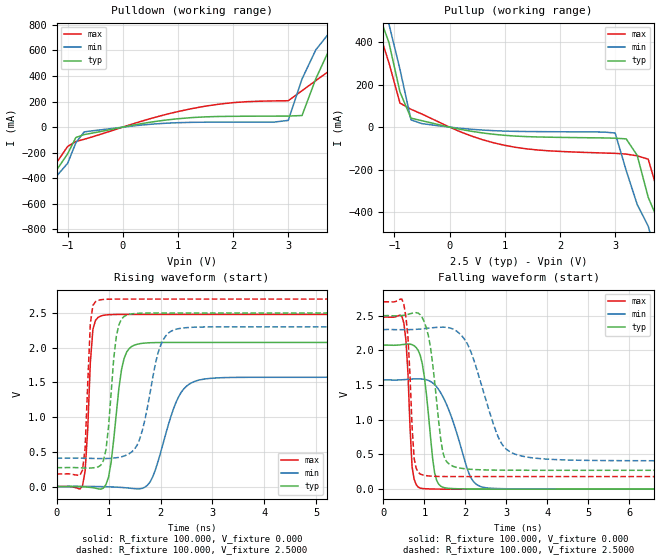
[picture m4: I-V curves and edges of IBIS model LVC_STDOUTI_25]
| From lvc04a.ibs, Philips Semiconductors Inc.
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|   Model LVC_STDOUTI_25
[Model]   LVC_STDOUTI_25
Model_type   Output
Polarity   Inverting
Vmeas =   1.25000V
Cref  =  50.0000pF
Rref  =   0.5000k
Vref  =   0.000V
C_comp   2.82pF   1.84pF   3.60pF
[Model Spec]
| Note: The input and output voltage ratings may be exceeded if the input and
|   output current ratings are observed (please refer to the data sheet)
|   Subparameter   typ   min   max
| Timing Thresholds
Vmeas   1.25   1.15   1.5
|Ambient temperature:   25.0000   85.0000   -40.0000
[Temperature Range]   35.0000   95.0000   -30.0000
[Voltage Range]   2.5000V   2.3000V   2.7000V
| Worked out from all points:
|   slope of the pulldown table from 0 to 0.375 V, typ, clamps not added: 12.6 ohm
|   slope of the pullup table from 0 to 0.375 V, typ, clamps not added: 20.2 ohm
|   rising waveform, R_fixture 100.000, V_fixture 0.000: 20-80 % time 185ps typ, 394ps min, 98.4ps max; typ from 0 V to 2.08 V
|   rising waveform, R_fixture 100.000, V_fixture 2.5000: 20-80 % time 154ps typ, 309ps min, 84.4ps max; typ from 0.272 V to 2.5 V
|   falling waveform, R_fixture 100.000, V_fixture 0.000: 20-80 % time 220ps typ, 524ps min, 118ps max; typ from 2.08 V to 0 V
|   falling waveform, R_fixture 100.000, V_fixture 2.5000: 20-80 % time 253ps typ, 608ps min, 125ps max; typ from 2.5 V to 0.272 V
|Process Range   nominal   slow   fast
[Pulldown]
| voltage   I(typ)   I(min)   I(max)
-5.5V     -4.532A    -4.567A    -4.49A
-1.75V    -813.8mA   -856.7mA   -763.9mA
-1.3V     -390.7mA   -435.2mA   -340.4mA
-850mV    -81.4mA    -123mA     -112.1mA
-700mV    -58.27mA   -37.32mA   -95.26mA
200mV     16.69mA    10.05mA    27.75mA
3V        86.6mA     52.68mA    206.7mA
3.25V     91mA       377.6mA    285.4mA
3.75V     613.8mA    741.2mA    442.7mA
4V        770.2mA    946.7mA    688.1mA
4.25V     1.002A     1.194A     872.6mA
11V       7.619A     7.847A     7.414A
[Pullup]
| voltage   I(typ)   I(min)   I(max)
-8.7V     7.804A     7.84A      7.774A
-1.5V     656.4mA    713.2mA    592mA
-1.3V     543.6mA    611.5mA    467mA
-1.1V     399.2mA    486.5mA    303.6mA
-900mV    166.1mA    272.9mA    113.6mA
-700mV    42.51mA    34.1mA     84.13mA
1V        -38.66mA   -18.69mA   -85.87mA
3V        -52.12mA   -27.61mA   -123.7mA
3.4V      -133.2mA   -364.8mA   -135.4mA
3.6V      -331.1mA   -467.1mA   -151.1mA
4V        -646.9mA   -851.8mA   -476.4mA
8.2V      -4.738A    -4.969A    -4.506A
[Ramp]
| variable   typ   min   max
dV/dt_r   1.245V/185.537ps   944.187mV/394.115ps   1.487V/98.353ps
dV/dt_f   1.337V/253.184ps   1.135V/608.079ps   1.511V/125.252ps
R_load = 100.000
[Rising Waveform]
R_fixture   = 100.000
V_fixture   = 0.000
V_fixture_min = 0.000
V_fixture_max = 0.000
| time   V(typ)   V(min)   V(max)
0s        41.03pV    1.687nV    3.181pV
500ps     -2.657mV   1.113mV    10.55mV
550ps     -5.724mV   1.075mV    224.8mV
700ps     -17.94mV   503.1uV    2.265V
850ps     -38.14mV   -1.361mV   2.456V
1ns       133.2mV    -4.473mV   2.475V
1.3ns     1.846V     -16.07mV   2.479V
1.55ns    2.049V     -33.74mV   2.479V
2.75ns    2.075V     1.535V     2.479V
9.75ns    2.075V     1.574V     2.479V
[Rising Waveform]
R_fixture   = 100.000
V_fixture   = 2.5000
V_fixture_min = 2.3000
V_fixture_max = 2.7000
| time   V(typ)   V(min)   V(max)
0s        272mV      409mV      181.2mV
500ps     267.4mV    408.1mV    236.4mV
550ps     265.6mV    407.2mV    553.4mV
650ps     266mV      405.3mV    2.343V
800ps     282.5mV    402.8mV    2.681V
950ps     525.6mV    403.1mV    2.697V
1.15ns    2.163V     414.3mV    2.7V
1.35ns    2.469V     454.2mV    2.7V
2.3ns     2.5V       2.265V     2.7V
9.75ns    2.5V       2.3V       2.7V
[Falling Waveform]
R_fixture   = 100.000
V_fixture   = 0.000
V_fixture_min = 0.000
V_fixture_max = 0.000
| time   V(typ)   V(min)   V(max)
0s        2.075V     1.574V     2.479V
500ps     2.085V     1.578V     2.39V
600ps     2.091V     1.582V     1.662V
700ps     2.082V     1.587V     323.7mV
900ps     1.927V     1.589V     15.62mV
1.25ns    236.3mV    1.507V     1.788mV
1.45ns    28.22mV    1.334V     594.9uV
2.1ns     2.591mV    210.8mV    18.13uV
2.4ns     1.124mV    32.77mV    3.651uV
9.75ns    48.02pV    641.2nV    3.182pV
[Falling Waveform]
R_fixture   = 100.000
V_fixture   = 2.5000
V_fixture_min = 2.3000
V_fixture_max = 2.7000
| time   V(typ)   V(min)   V(max)
0s        2.5V       2.3V       2.7V
500ps     2.505V     2.297V     2.661V
600ps     2.518V     2.298V     2.186V
750ps     2.541V     2.301V     444.7mV
900ps     2.513V     2.307V     217.5mV
1.15ns    2.043V     2.324V     188.4mV
1.45ns    535.1mV    2.334V     182.5mV
1.7ns     329.9mV    2.307V     181.5mV
3.2ns     272.7mV    507.2mV    181.2mV
9.75ns    272mV      409mV      181.2mV
